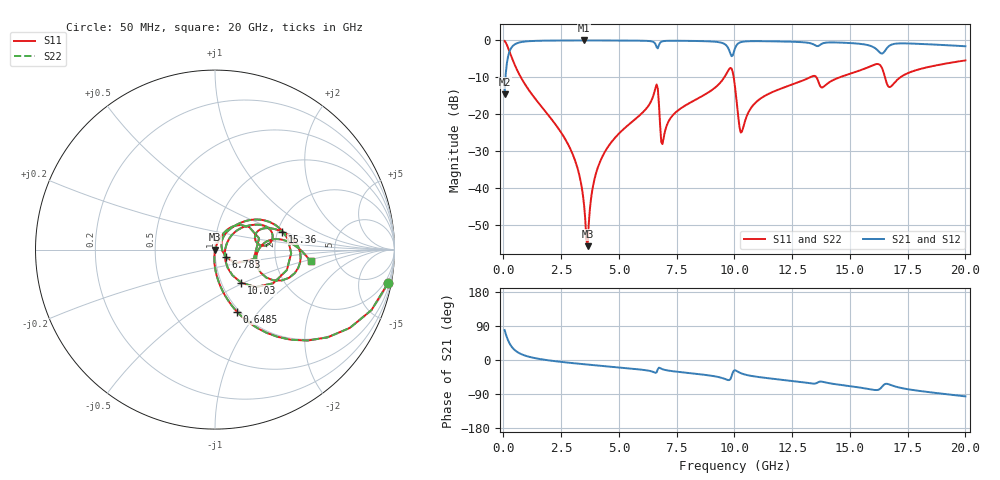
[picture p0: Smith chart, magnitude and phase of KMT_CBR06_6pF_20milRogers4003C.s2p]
! Data measured by Modelithics Inc. support@modelithics.com 813-866-6335
! KEMET CBR0603 6pF, Pad Width= 0.851mm, Pad Length= 0.64mm, Pad Gap= 0.62mm, 20mil Rogers 4003C substrate Data, January 2022
# hz S ma R 50
! 2 Port Network Data from SP1.SP block
! freq  magS11  angS11  magS21  angS21  magS12  angS12  magS22  angS22
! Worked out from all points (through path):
!   401 points, 50 MHz to 20 GHz, reference 50 ohm
!   highest |S21| = -0.01 dB at 3.491 GHz (marker M1); lowest = -14.6 dB at 50 MHz (marker M2)
!   group delay of S21, straight-line fit = 14.8 ps
!   lowest |S11| = -55.7 dB at 3.641 GHz (marker M3), VSWR 1.00, Z = 50.2 + j0.043 ohm
!   |S11| at or under -10 dB: 755.9 MHz to 9.561 GHz (8.805 GHz wide, 171 % of centre); 9.969 GHz to 13.27 GHz (3.298 GHz wide, 28.4 % of centre); 13.55 GHz to 14.55 GHz (998.8 MHz wide, 7.11 % of centre)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
!   |S22| runs from -55.7 to -0.2 dB; largest |S21 - S12| = 0
!   S11 on the Smith chart (normalised r, x): 50 MHz: 1, -10; 648.5 MHz: 0.97, -0.77; 6.783 GHz: 1.12, -0.09; 10.03 GHz: 1.24, -0.48; 15.36 GHz: 2.11, +0.50; 20 GHz: 3.19, -0.59
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5e7  0.9823 -10.9  0.1868 79.1  0.1868 79.1  0.9823 -10.9
2.495e8  0.7236 -44.4  0.6897 45.5  0.6897 45.5  0.7236 -44.4
6.485e8  0.3657 -70.6  0.93 19.3  0.93 19.3  0.3657 -70.6
2.74325e9  0.04229 -94.9  0.9977 -6.6  0.9977 -6.6  0.04229 -94.9
3.391625e9  0.01023 -92.7  0.9984 -10.6  0.9984 -10.6  0.01023 -92.7
3.491375e9  0.005882 -87.1  0.9984 -11.2  0.9984 -11.2  0.005882 -87.1
3.641e9  0.001648 15.1  0.9984 -12.1  0.9984 -12.1  0.001648 15.1
3.94025e9  0.01324 69.6  0.9982 -13.8  0.9982 -13.8  0.01324 69.6
4.439e9  0.03292 70.6  0.9976 -16.5  0.9976 -16.5  0.03292 70.6
6.583625e9  0.2284 33.3  0.8886 -33.8  0.8886 -33.8  0.2284 33.3
6.73325e9  0.1352 -34.2  0.868 -20.2  0.868 -20.2  0.1352 -34.2
6.783125e9  0.07114 -34.1  0.9303 -21.4  0.9303 -21.4  0.07114 -34.1
6.93275e9  0.04783 40.9  0.9795 -25.3  0.9795 -25.3  0.04783 40.9
9.476375e9  0.2897 35.4  0.9224 -47.7  0.9224 -47.7  0.2897 35.4
1.0025e10  0.2359 -51.5  0.7801 -27.1  0.7801 -27.1  0.2359 -51.5
1.032425e10  0.05828 6.1  0.9556 -35.9  0.9556 -35.9  0.05828 6.1
1.107238e10  0.1587 41.2  0.9768 -45.1  0.9768 -45.1  0.1587 41.2
1.336662e10  0.3268 19.8  0.8998 -62.1  0.8998 -62.1  0.3268 19.8
1.536162e10  0.3857 15.2  0.9037 -72.1  0.9037 -72.1  0.3857 15.2
1.625938e10  0.475 -12.4  0.7038 -77.8  0.7038 -77.8  0.475 -12.4
1.670825e10  0.2333 -9.9  0.846 -64.5  0.846 -64.5  0.2333 -9.9
2e10  0.5364 -7.1  0.833 -96.0  0.833 -96.0  0.5364 -7.1
